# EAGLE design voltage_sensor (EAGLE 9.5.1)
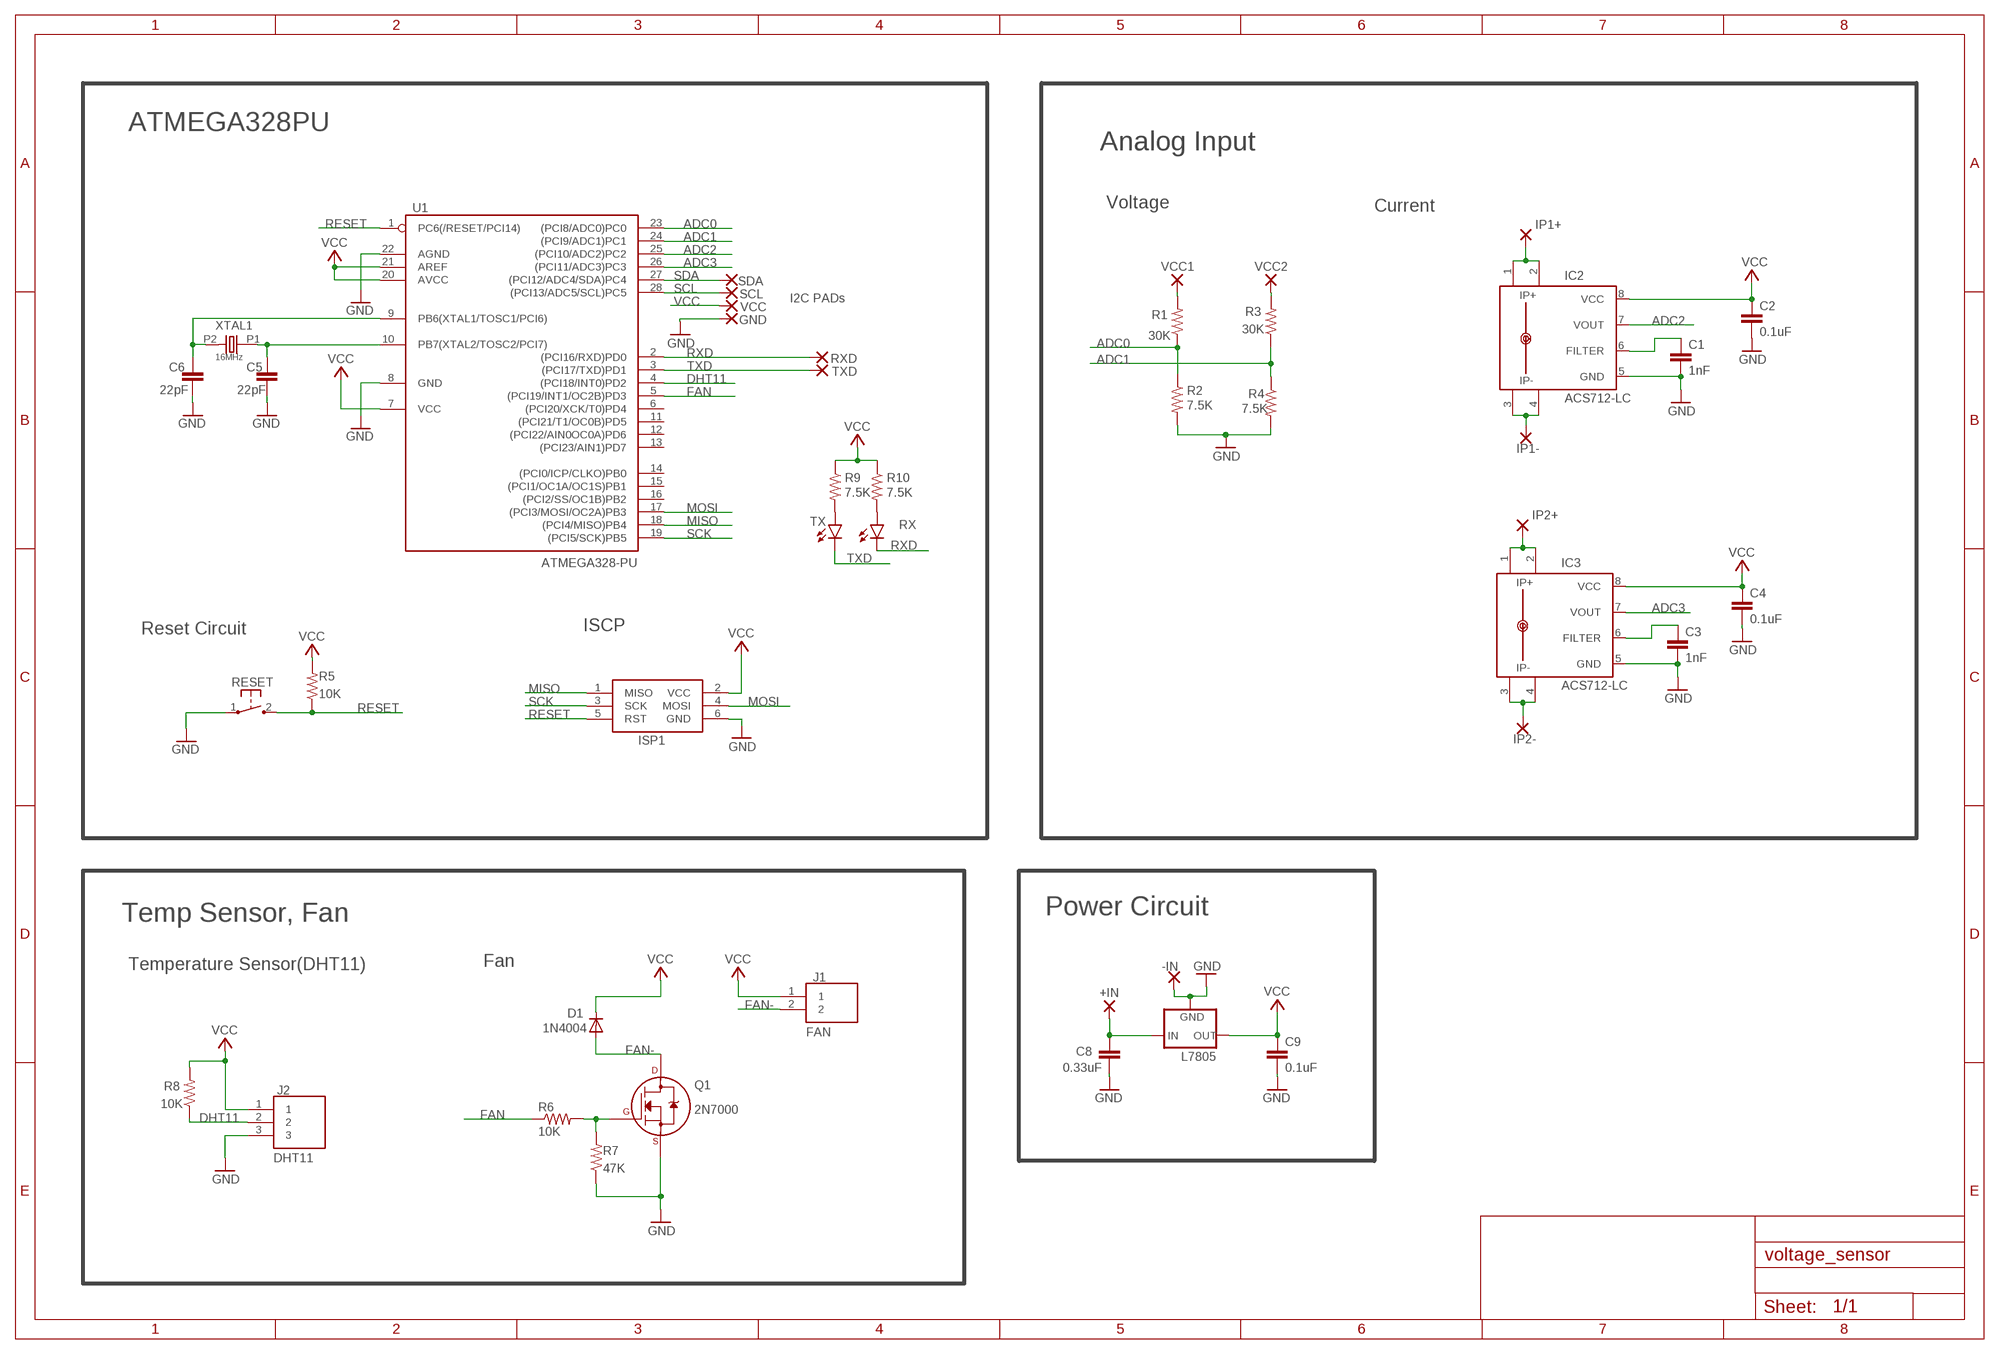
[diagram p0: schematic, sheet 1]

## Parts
+IN  1,6/0,8  [1,6/0,8]
-IN  1,6/0,8  [1,6/0,8]
C1  1nF  C2,5-3  [C2.5-3]
C2  0.1uF  C2,5-3  [C2.5-3]
C3  1nF  C2,5-3  [C2.5-3]
C4  0.1uF  C2,5-3  [C2.5-3]
C5  22pF  C2,5-3  [C2.5-3]
C6  22pF  C2,5-3  [C2.5-3]
C8  0.33uF  C2,5-3  [C2.5-3]
C9  0.1uF  C2,5-3  [C2.5-3]
D1  1N4004  [DO41-10]
GND  GND  1,6/0,8  [1,6/0,8]
IC2  ACS712-LC  [SOIC8]
IC3  ACS712-LC  [SOIC8]
IP1+  1,6/0,8  [1,6/0,8]
IP1-  1,6/0,8  [1,6/0,8]
IP2+  1,6/0,8  [1,6/0,8]
IP2-  1,6/0,8  [1,6/0,8]
ISP1  AVRISP-6  [AVRISP]
J1  FAN  B2B-PH-K-S_LF__SN_  [SHDR2W50P0X200_1X2_590X450X600]
J2  DHT11  B3B-PH-K-S_LF__SN_  [SHDR3W50P0X200_1X3_790X450X600]
L7805  78XXS  [78XXS]
Q1  2N7000  2N7000_TO92  [TO-92]
R1  30K  R-US_0204/2V  [0204V]
R2  7.5K  R-US_0204/2V  [0204V]
R3  30K  R-US_0204/2V  [0204V]
R4  7.5K  R-US_0204/2V  [0204V]
R5  10K  R-US_0204/2V  [0204V]
R6  10K  R-US_0204/2V  [0204V]
R7  47K  R-US_0204/2V  [0204V]
R8  10K  R-US_0204/2V  [0204V]
R9  7.5K  R-US_0204/2V  [0204V]
R10  7.5K  R-US_0204/2V  [0204V]
RESET  3X4X2_2PIN_SWITCH  [33X4X2_2PIN_SWITCH]
RX  LED3MM  [LED3MM]
RXD  RXD  1,6/0,8  [1,6/0,8]
SCL  1,6/0,8  [1,6/0,8]
SDA  1,6/0,8  [1,6/0,8]
TX  LED3MM  [LED3MM]
TXD  GND  1,6/0,8  [1,6/0,8]
U1  ATMEGA328-PU  ATMEGA168-20P  [DIL28-3]
VCC  1,6/0,8  [1,6/0,8]
VCC1  1,6/0,8  [1,6/0,8]
VCC2  1,6/0,8  [1,6/0,8]
XTAL1  16MHz  OSC-XTAL-HC-49U-PTH  [HC-49U-PTH]

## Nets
+IN: +IN.1(P) C8.2 L7805.IN
ADC0: R1.1 R2.1 U1.23((PCI8/ADC0)PC0)
ADC1: R3.1 R4.1 U1.24((PCI9/ADC1)PC1)
ADC2: IC2.7(VOUT) U1.25((PCI10/ADC2)PC2)
ADC3: IC3.7(VOUT) U1.26((PCI11/ADC3)PC3)
DHT11: J2.2 R8.1 U1.4((PCI18/INT0)PD2)
FAN: R6.1 U1.5((PCI19/INT1/OC2B)PD3)
FAN-: D1.A J1.2 Q1.3(D)
GND: -IN.1(P) C1.2 C2.2 C3.2 C4.2 C5.1 C6.1 C8.1 C9.2 GND.1(P) IC2.5(GND) IC3.5(GND) ISP1.6(GND) J2.3 L7805.GND Q1.1(S) R2.2 R4.2 R7.1 RESET.1(P) U1.8(GND) U1.22(AGND)
IP1+: IC2.1(IP+) IC2.2(IP+1) IP1+.1(P)
IP1-: IC2.3(IP-) IC2.4(IP-1) IP1-.1(P)
IP2+: IC3.1(IP+) IC3.2(IP+1) IP2+.1(P)
IP2-: IC3.3(IP-) IC3.4(IP-1) IP2-.1(P)
MISO: ISP1.1(MISO) U1.18((PCI4/MISO)PB4)
MOSI: ISP1.4(MOSI) U1.17((PCI3/MOSI/OC2A)PB3)
N$1: R1.2 VCC1.1(P)
N$2: R10.2 RX.A
N$3: C6.2 U1.9(PB6(XTAL1/TOSC1/PCI6)) XTAL1.P2
N$4: C5.2 U1.10(PB7(XTAL2/TOSC2/PCI7)) XTAL1.P1
N$5: R9.2 TX.A
N$7: C1.1 IC2.6(FILTER)
N$11: C3.1 IC3.6(FILTER)
N$24: Q1.2(G) R6.2 R7.2
RESET: ISP1.5(RST) R5.1 RESET.2(S) U1.1(PC6(/RESET/PCI14))
RXD: RX.K(C) RXD.1(P) U1.2((PCI16/RXD)PD0)
SCK: ISP1.3(SCK) U1.19((PCI5/SCK)PB5)
SCL: SCL.1(P) U1.28((PCI13/ADC5/SCL)PC5)
SDA: SDA.1(P) U1.27((PCI12/ADC4/SDA)PC4)
TXD: TX.K(C) TXD.1(P) U1.3((PCI17/TXD)PD1)
VCC: C2.1 C4.1 C9.1 D1.C IC2.8(VCC) IC3.8(VCC) ISP1.2(VCC) J1.1 J2.1 L7805.OUT R5.2 R8.2 R9.1 R10.1 U1.7(VCC) U1.20(AVCC) U1.21(AREF) VCC.1(P)
VCC2: R3.2 VCC2.1(P)
Unconnected: U1.6((PCI20/XCK/T0)PD4) U1.11((PCI21/T1/OC0B)PD5) U1.12((PCI22/AIN0OC0A)PD6) U1.13((PCI23/AIN1)PD7) U1.14((PCI0/ICP/CLKO)PB0) U1.15((PCI1/OC1A/OC1S)PB1) U1.16((PCI2/SS/OC1B)PB2)

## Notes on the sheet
- ATMEGA328PU
- Analog Input
- Voltage | Current
- I2C PADs
- Reset Circuit | ISCP
- Temp Sensor, Fan | Power Circuit
- Temperature Sensor(DHT11) | Fan

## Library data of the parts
+IN -IN GND IP1+ IP1- IP2+ IP2- RXD SCL SDA TXD VCC VCC1 VCC2 = wirepad:1,6/0,8: THROUGH-HOLE PAD
C1-C6 C8 C9 = capacitor-wima:C: CAPACITOR
D1 = adafruit:1N4004: DIODE
IC2 IC3 = allegro-2:ACS712-LC
ISP1 = adafruit:AVRISP: AVR ISP HEADER Standard 6 pin header for AVR programming
J1 = B2B-PH-K-S_LF__SN_:B2B-PH-K-S_LF__SN_: PH-2.0mm Header top entry 2 way JST PH Series, Series Number B2B, 2mm Pitch 2 Way 1 Row Straight PCB Header, Through Hole Termination, 2A; ARROW_PART_NUMBER: B2B-PH-K-S(LF)(SN); ARROW_PRICE-STOCK: https://www.arrow.com/en/products/b2b-ph-k-s-lf-sn/jst-manufacturing; DESCRIPTION: PH-2.0mm Header top entry 2 way JST PH Series, Series Number B2B, 2mm Pitch 2 Way 1 Row Straight PCB Header, Through Hole Termination, 2A; HEIGHT: 6mm; MANUFACTURER_NAME: JST (JAPAN SOLDERLESS TERMINALS); MANUFACTURER_PART_NUMBER: B2B-PH-K-S(LF)(SN)
J2 = B3B-PH-K-S_LF__SN_:B3B-PH-K-S_LF__SN_: PH-2.0mm Header top entry 3 way JST PH Series, Series Number B3B, 2mm Pitch 3 Way 1 Row Straight PCB Header, Through Hole Termination, 2A Source: Datasheet; ARROW_PART_NUMBER: B3B-PH-K-S(LF)(SN); ARROW_PRICE-STOCK: https://www.arrow.com/en/products/b3b-ph-k-s-lf-sn/jst-manufacturing; DESCRIPTION: PH-2.0mm Header top entry 3 way JST PH Series, Series Number B3B, 2mm Pitch 3 Way 1 Row Straight PCB Header, Through Hole Termination, 2A; HEIGHT: 6mm; MANUFACTURER_NAME: JST (JAPAN SOLDERLESS TERMINALS); MANUFACTURER_PART_NUMBER: B3B-PH-K-S(LF)(SN)
L7805 = v-reg:78XXS: VOLTAGE REGULATOR
Q1 = transistors:2N700*: 2N7000, 2N7002, NDS7002A N-channel enhancement mode MOSFET
R1-R10 = adafruit:R-US_: RESISTOR, American symbol
RESET = MyLib:3X4X2_2PIN_SWITCH
RX TX = led:LED: LED
U1 = adafruit:ATMEGA168*P: MICROCONTROLLER 16 kBytes FLASH 1 kBytes SRAM 512 Bytes EEPROM USART 8-channel 10 bit ADC
XTAL1 = dp_devices:OSC-XTAL

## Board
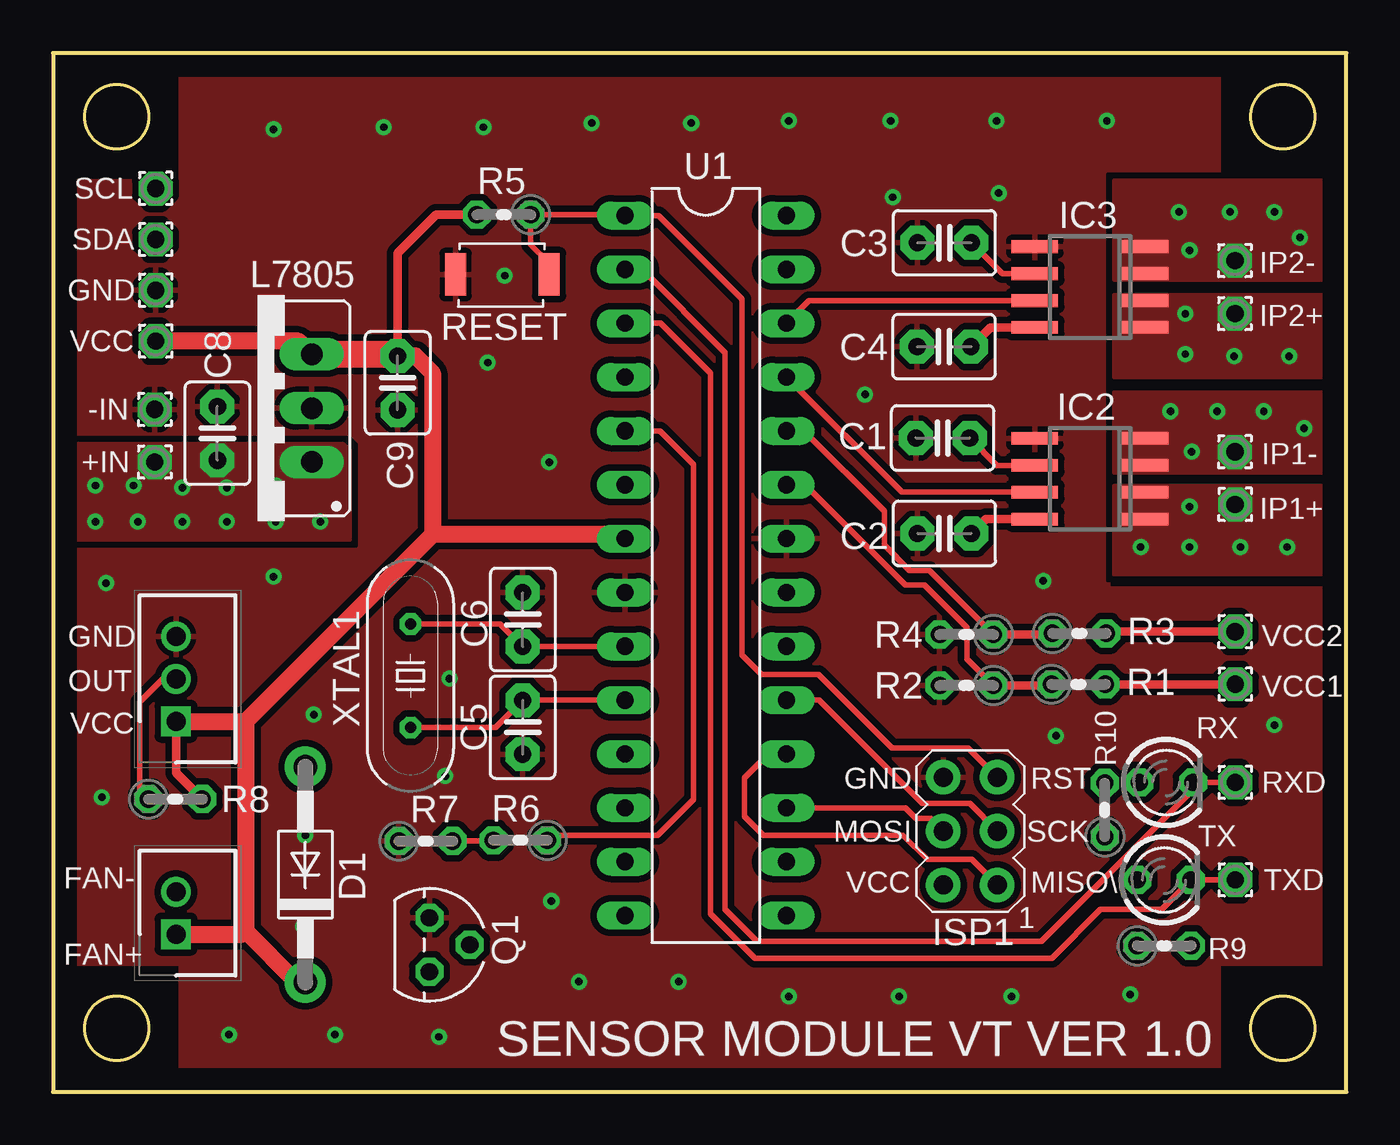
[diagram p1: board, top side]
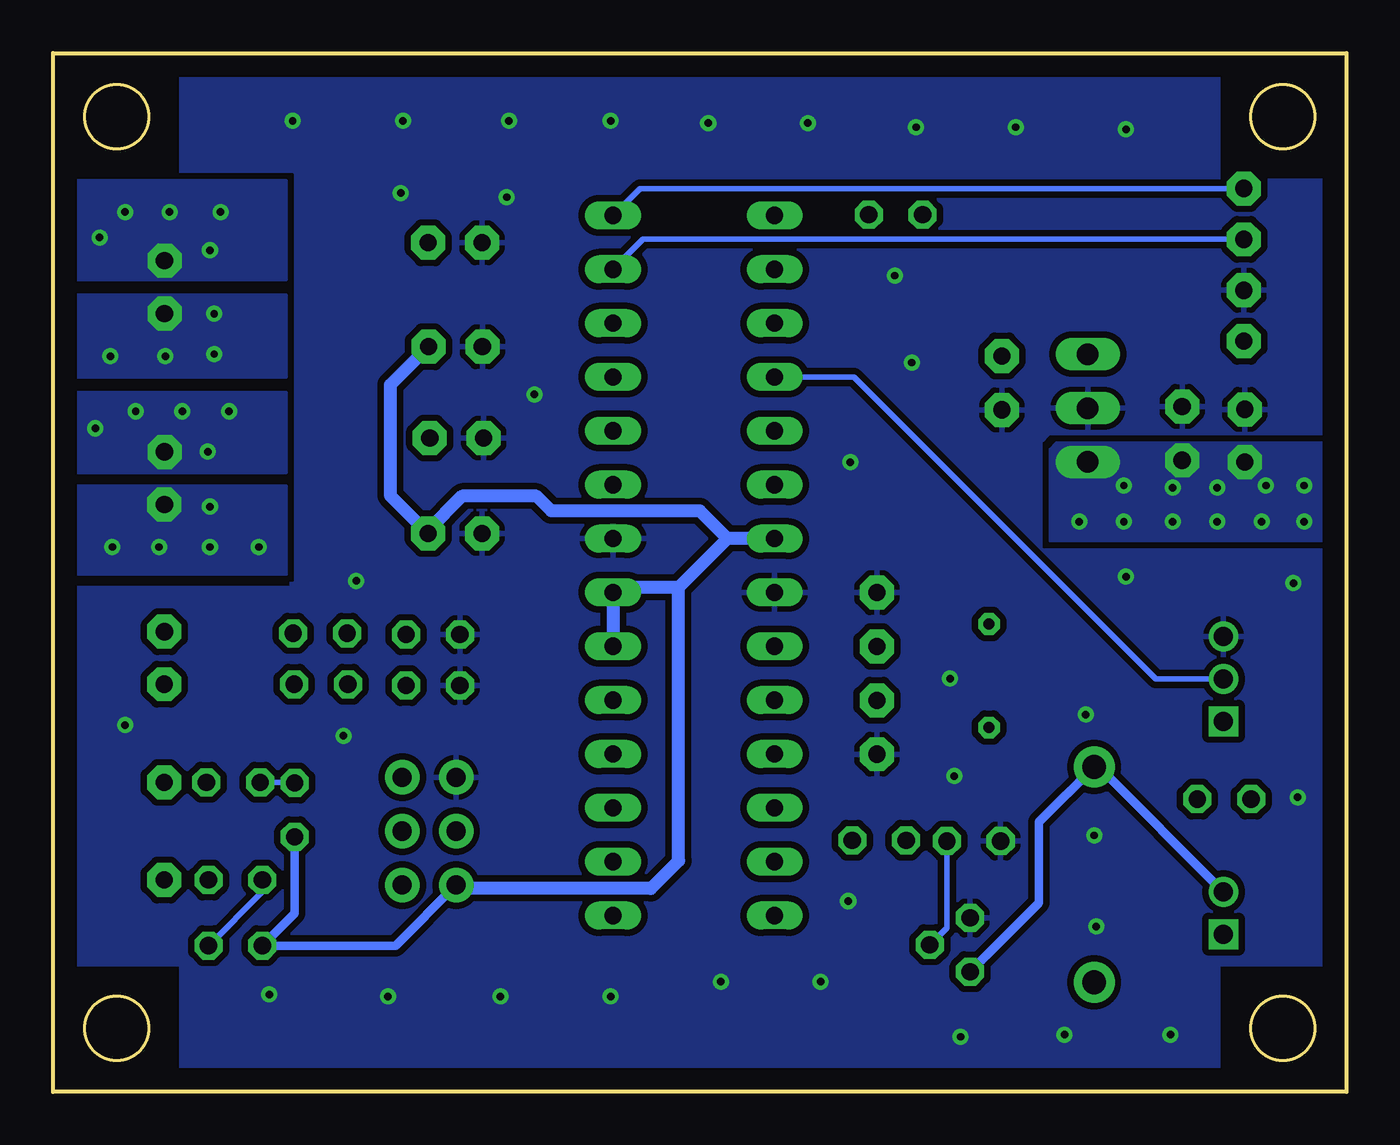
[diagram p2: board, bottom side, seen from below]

Size 61 x 49 mm. Coordinates in mm from the lower left corner, seen from the top.
Outline: 0,0 61,0 61,49 0,49 0,0
Outline: circle at 3,46 radius 1.5
Outline: circle at 3,3 radius 1.5
Outline: circle at 58,3 radius 1.5
Outline: circle at 58,46 radius 1.5
Copper layers (1*16): Top 0.035mm / dielectric 1.5mm / Bottom 0.035mm
Design rules "default": minimum track width 6mil, minimum drill 0.35mm, track to track 6mil, track to pad 6mil, pad to pad 6mil, via to via 6mil, smd to smd 6mil, copper to edge 40mil, drill to drill 6mil, minimum pad ring 10mil, minimum via ring 8mil, stop-mask expansion 4mil, vias tented up to drill 0mil, thermal gap 10mil

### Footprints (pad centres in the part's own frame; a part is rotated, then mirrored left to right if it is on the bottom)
1,6/0,8 = drill 0.813 pad 1.6 octagon: 1 0,0
C2.5-3 = drill 0.813 pad 1.6 octagon: 1 -1.27,0; 2 1.27,0
DO41-10 = drill 1.118 pad 1.93: A 5.08,0; C -5.08,0
SOIC8 = smd 0.6 x 2.2: 1 -1.905,-2.6; 2 -0.635,-2.6; 3 0.635,-2.6; 4 1.905,-2.6; 5 1.905,2.6; 6 0.635,2.6; 7 -0.635,2.6; 8 -1.905,2.6
AVRISP = drill 0.9 pad 1.626: 1 -1.27,2.54; 2 1.27,2.54; 3 -1.27,0; 4 1.27,0; 5 -1.27,-2.54; 6 1.27,-2.54
SHDR2W50P0X200_1X2_590X450X600 = drill 0.9 pad 1.35 square: 1 0,0 | drill 0.9 pad 1.35: 2 -2,0
SHDR3W50P0X200_1X3_790X450X600 = drill 0.9 pad 1.35 square: 1 0,0 | drill 0.9 pad 1.35: 2 -2,0; 3 -4,0
78XXS = drill 1.016 long: GND 0,-2.54; IN -2.54,-2.54; OUT 2.54,-2.54
TO-92 = drill 0.813 octagon: 1 -1.27,0; 2 0,1.905; 3 1.27,0
0204V = drill 0.813 octagon: 1 -1.27,0; 2 1.27,0
33X4X2_2PIN_SWITCH = smd 1 x 2: 1 -2.2,0; 2 2.2,0
LED3MM = drill 0.813 octagon: A -1.27,0; K 1.27,0
DIL28-3 = drill 0.813 long: 1 -16.51,-3.81; 2 -13.97,-3.81; 3 -11.43,-3.81; 4 -8.89,-3.81; 5 -6.35,-3.81; 6 -3.81,-3.81; 7 -1.27,-3.81; 8 1.27,-3.81; 9 3.81,-3.81; 10 6.35,-3.81; 11 8.89,-3.81; 12 11.43,-3.81; 13 13.97,-3.81; 14 16.51,-3.81; 15 16.51,3.81; 16 13.97,3.81; 17 11.43,3.81; 18 8.89,3.81; 19 6.35,3.81; 20 3.81,3.81; 21 1.27,3.81; 22 -1.27,3.81; 23 -3.81,3.81; 24 -6.35,3.81; 25 -8.89,3.81; 26 -11.43,3.81; 27 -13.97,3.81; 28 -16.51,3.81
HC-49U-PTH = drill 0.508 octagon: P1 -2.44,0; P2 2.44,0

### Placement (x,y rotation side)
+IN  4.8,29.71 0 top
-IN  4.8,32.19 0 top
C1  41.96,30.84 180 top
C2  42.04,26.34 180 top
C3  42.04,40.05 180 top
C4  42.02,35.15 180 top
C5  22.15,17.2 90 top
C6  22.15,22.28 270 top
C8  7.75,31.06 270 top
C9  16.25,33.44 270 top
D1  11.9,10.25 90 top
GND  4.84,37.81 0 top
IC2  48.9,28.92 90 top
IC3  48.9,37.96 90 top
IP1+  55.75,27.71 0 top
IP1-  55.74,30.19 0 top
IP2+  55.74,36.71 0 top
IP2-  55.74,39.21 0 top
ISP1  43.26,12.3 180 top
J1  5.8,7.44 270 top
J2  5.8,17.48 270 top
L7805  9.66,32.25 90 top
Q1  17.75,6.94 270 top
R1  48.36,19.23 0 top
R2  43.08,19.17 180 top
R3  48.4,21.63 0 top
R4  43.08,21.57 180 top
R5  21.26,41.37 180 top
R6  22.04,11.87 180 top
R7  17.58,11.83 0 top
R8  5.77,13.81 0 top
R9  52.4,6.9 0 top
R10  49.6,13.3 90 top
RESET  21.19,38.55 0 top
RX  52.5,14.6 0 top
RXD  55.76,14.6 0 top
SCL  4.84,42.61 0 top
SDA  4.84,40.21 0 top
TX  52.4,10 0 top
TXD  55.76,10 0 top
U1  30.78,24.83 270 top
VCC  4.84,35.41 0 top
VCC1  55.76,19.23 0 top
VCC2  55.75,21.71 0 top
XTAL1  16.86,19.63 90 top

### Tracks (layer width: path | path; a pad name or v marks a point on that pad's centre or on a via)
+IN  (via drill 0.35)
  other vias: 2,28.6 2,26.9 4,26.9 6.1,26.9 8.2,26.9 10.5,26.9 12.6,26.9 6.1,28.5 10.5,28.6 8.2,28.5 3.8,28.6
  pour Top (isolate 0.305, no thermals): 0,30.6 13.7,30.6 14,30.3 14,26 0,26
  pour Bottom (isolate 0.305, no thermals): 0,30.6 13.7,30.6 14,30.3 14,26 0,26
ADC0
  Top 0.254: U1.23 35.46,28.64 40.2,23.9 41.1,23.9 43.1,21.9 43.1,20.42 R2.1
  Top 0.406: R2.1 47.03,19.17 R1.1
ADC1
  Top 0.254: R4.1 41.32,24.6 40.4,24.6 39.2,25.8 39.2,27.4 35.42,31.18 U1.24
  Top 0.406: R4.1 47.07,21.57 R3.1
ADC2
  Top 0.254: IC2.7 40.02,28.29 U1.25
ADC3
  Top 0.254: IC3.7 35.66,37.33 U1.26
DHT11
  Top 0.254: R8.1 4.1,14.21 4.1,18.4 5.18,19.48 J2.2
  Bottom 0.254: J2.2 8.98,19.48 23.22,33.72 U1.4
FAN
  Top 0.254: U1.5 28.62,31.18 30.2,29.6 30.2,13.8 28.5,12.1 23.54,12.1 R6.1
FAN-
  Bottom 0.406: J1.2 11.69,15.33 D1.A 14.5,12.73 14.5,8.92 Q1.3
GND  (via drill 0.35)
  other vias: 24.8,5.2 29.5,5.2 23.5,9 34.7,4.5 39.9,4.5 45.2,4.5 50.8,4.6 47.3,16.8 18.2,2.6 13.3,2.7 11.9,12.1 11.8,7.8 8.3,2.7 10.4,24.3 12.3,17.8 2.3,13.9 2.5,24 18.7,19.5 18.5,14.9 23.4,29.7 20.5,34.4 10.4,45.4 15.6,45.5 20.3,45.5 25.4,45.7 30.1,45.7 34.7,45.8 39.5,45.8 44.5,45.8 49.7,45.8 44.6,42.4 39.6,42.2 21.3,38.5 38.3,32.9 46.7,24.1 57.6,17.3
  pour Top (isolate 0.305, rank 2): 6,0 6,6 0,6 0,43 6,43 6,49 55,49 55,43 49.8,43 49.8,23.8 61,23.8 61,6 55,6 55,0
  pour Bottom (isolate 0.305, rank 2): 6,0 6,6 0,6 0,43 6,43 6,49 55,49 55,43 49.8,43 49.8,23.8 61,23.8 61,6 55,6 55,0
IP1+  (via drill 0.35)
  other vias: 53.6,27.6 51.3,25.7 53.6,25.7 56,25.7 58.2,25.7
  pour Top (isolate 0.305, no thermals): 61,28.6 50,28.6 50,24.4 61,24.4
  pour Bottom (isolate 0.305, no thermals): 61,28.6 50,28.6 50,24.4 61,24.4
IP1-  (via drill 0.35)
  other vias: 52.7,32.1 54.9,32.1 57.1,32.1 59,31.3 53.7,30.2
  pour Top (isolate 0.305, no thermals): 61,33 50,33 50,29.2 61,29.2
  pour Bottom (isolate 0.305, no thermals): 61,33 50,33 50,29.2 61,29.2
IP2+  (via drill 0.35)
  other vias: 53.4,36.7 53.4,34.8 55.7,34.7 58.3,34.7
  pour Top (isolate 0.305, no thermals): 61,37.6 50,37.6 50,33.7 61,33.7
  pour Bottom (isolate 0.305, no thermals): 61,37.6 50,37.6 50,33.7 61,33.7
IP2-  (via drill 0.35)
  other vias: 57.6,41.5 58.8,40.3 53.1,41.5 53.6,39.7 55.5,41.5
  pour Bottom (isolate 0.305, no thermals): 61,43 50,43 50,38.3 61,38.3
  pour Top (isolate 0.305, no thermals): 61,43 50,43 50,38.3 61,38.3
MISO
  Top 0.254: ISP1.1 43.33,10.96 41.23,10.96 40.09,12.1 33.5,12.1 32.6,13 32.6,14.8 33.74,15.94 U1.18
MOSI
  Top 0.254: ISP1.4 41.39,12.9 40.69,12.9 40.19,13.4 U1.17
N$1
  Top 0.406: VCC1.1 R1.2
N$2
  Bottom 0.254: R10.2 49.63,14.6 RX.A
N$3
  Top 0.254: XTAL1.P2 21.09,22.07 C6.2 U1.9
N$4
  Top 0.254: U1.10 C5.2 20.87,17.19 XTAL1.P1
N$5
  Bottom 0.254: R9.2 51.13,9.44 TX.A
N$7
  Top 0.254: IC2.6 44.52,29.55 C1.1
N$11
  Top 0.254: IC3.6 44.77,38.59 C3.1
N$24
  Top 0.254: R7.2 20.73,11.83 R6.2
  Bottom 0.254: Q1.2 18.85,7.75 R7.2
RESET
  Top 0.254: RESET.2 23.39,39.11 22.53,39.97 R5.1 26.94,41.37 U1.1 28.56,41.34 32.5,37.4 32.5,20.6 33.4,19.7 36.1,19.7 39.56,16.23 43.13,16.23 ISP1.5
RXD
  Top 0.254: U1.2 27.77,38.8 31.7,34.87 31.7,8.6 33.2,7.1 46.6,7.1 53.77,14.27 RX.K RXD.1
SCK
  Top 0.254: U1.19 36.12,18.48 41,13.6 43.23,13.6 ISP1.3
SCL
  Bottom 0.254: SCL.1 33.32,42.61 U1.28
SDA
  Bottom 0.254: SDA.1 33.18,40.21 U1.27
TXD
  Top 0.254: U1.3 28.64,36.26 31,33.9 31,8.4 33.1,6.3 47.1,6.3 49.4,8.6 52.3,8.6 53.67,9.97 TX.K TXD.1
VCC
  Top 0.406: IC3.8 44.2,36.05 C4.1 | IC2.8 43.98,27.02 C2.1 | C9.1 16.25,39.55 18.07,41.37 R5.2 | R8.2 5.8,15.05 J2.1
  Top 0.813: L7805.OUT 11.58,35.41 VCC.1 | J2.1 9.08,17.48 | 9.08,17.48 9.08,7.59 | C9.1 17.09,34.71 17.9,33.9 17.9,26.3 | 17.9,26.3 9.08,17.48 | U1.7 26.77,26.3 17.9,26.3 | D1.C 11.5,5.17 9.08,7.59 | J1.1 8.93,7.44 9.08,7.59
  Top 1.27: L7805.OUT 16.17,34.79 C9.1
  Bottom 0.406: ISP1.2 44.85,6.9 R9.1 49.6,8.43 R10.1
  Bottom 0.61: U1.7 29.2,26.1 | 29.2,26.1 30.5,27.4 37.5,27.4 38.2,28.1 41.7,28.1 43.31,26.49 C2.1 45.1,28.13 45.1,33.34 C4.1 | 29.2,26.1 31.5,23.8 | ISP1.2 41.83,9.6 32.8,9.6 31.5,10.9 31.5,23.8 | 31.5,23.8 34.35,23.8 U1.21 U1.20
VCC2
  Top 0.406: VCC2.1 49.75,21.71 R3.2

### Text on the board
tPlace: GND | OUT | VCC | GND | RST | MOSI | SCK | FAN- | VCC | MISO\ | FAN+ | SENSOR MODULE VT VER 1.0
